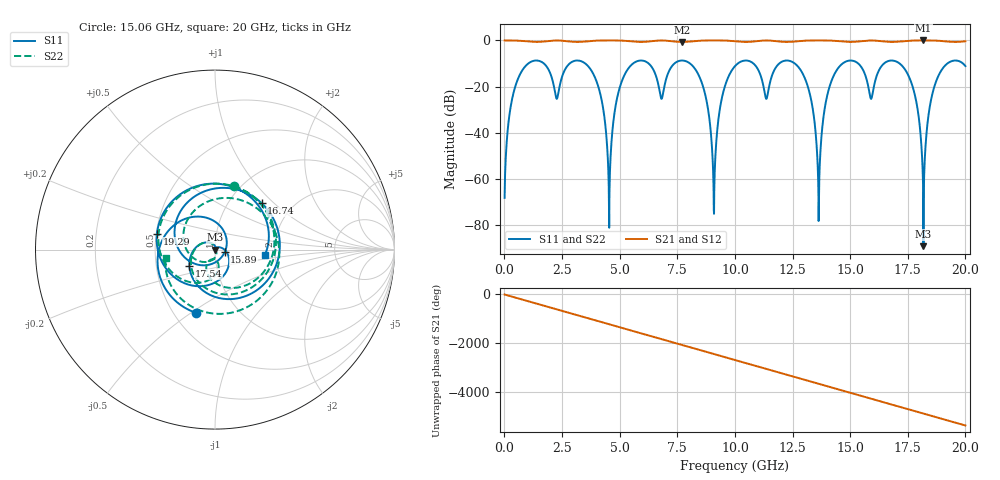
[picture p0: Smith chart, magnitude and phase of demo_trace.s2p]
! Created with skrf 1.12.0 (http://scikit-rf.org).
# GHz S RI R 50.0
!freq ReS11 ImS11 ReS21 ImS21 ReS12 ImS12 ReS22 ImS22
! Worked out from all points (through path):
!   2001 points, 10 MHz to 20 GHz, reference 50 ohm
!   highest |S21| = 0.00 dB at 18.18 GHz (marker M1); lowest = -0.6 dB at 7.706 GHz (marker M2)
!   group delay of S21, straight-line fit = 750 ps
!   lowest |S11| = -89.0 dB at 18.18 GHz (marker M3), VSWR 1.00, Z = 50 - j0.00142 ohm
!   |S11| at or under -10 dB: 3.512 GHz to 5.579 GHz (2.066 GHz wide, 45.5 % of centre); 12.6 GHz to 14.67 GHz (2.066 GHz wide, 15.2 % of centre); 17.15 GHz to 19.22 GHz (2.067 GHz wide, 11.4 % of centre)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
!   |S22| runs from -89.0 to -8.7 dB; largest |S21 - S12| = 7e-16
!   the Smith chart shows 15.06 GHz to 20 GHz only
!   S11 on the Smith chart (normalised r, x): 15.06 GHz: 0.64, -0.52; 15.89 GHz: 1.11, -0.03; 16.74 GHz: 1.41, +0.84; 17.54 GHz: 0.74, -0.14; 19.29 GHz: 0.50, +0.10; 20 GHz: 1.76, -0.12
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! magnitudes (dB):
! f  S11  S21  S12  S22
! 10 MHz  -68.1  0.0  0.0  -68.1
! 789.6 MHz  -12.7  -0.2  -0.2  -12.7
! 3.348 GHz  -9.0  -0.6  -0.6  -9.0
! 4.118 GHz  -21.5  0.0  0.0  -21.5
! 4.548 GHz  -81.1  0.0  0.0  -81.1
! 5.307 GHz  -13.2  -0.2  -0.2  -13.2
! 6.677 GHz  -19.0  -0.1  -0.1  -19.0
! 7.706 GHz  -8.7  -0.6  -0.6  -8.7
! 8.616 GHz  -19.8  0.0  0.0  -19.8
! 9.085 GHz  -73.5  0.0  0.0  -73.5
! 10.01 GHz  -11.1  -0.3  -0.3  -11.1
! 13.34 GHz  -27.5  0.0  0.0  -27.5
! 13.64 GHz  -71.5  0.0  0.0  -71.5
! 14.12 GHz  -19.5  0.0  0.0  -19.5
! 15.06 GHz  -8.7  -0.6  -0.6  -8.7
! 15.89 GHz  -25.1  0.0  0.0  -25.1
! 16.67 GHz  -8.9  -0.6  -0.6  -8.9
! 16.74 GHz  -8.7  -0.6  -0.6  -8.7
! 17.54 GHz  -15.5  -0.1  -0.1  -15.5
! 18.18 GHz  -89.0  0.0  0.0  -89.0
! 19.29 GHz  -9.5  -0.5  -0.5  -9.5
! 20 GHz  -11.1  -0.4  -0.4  -11.1
